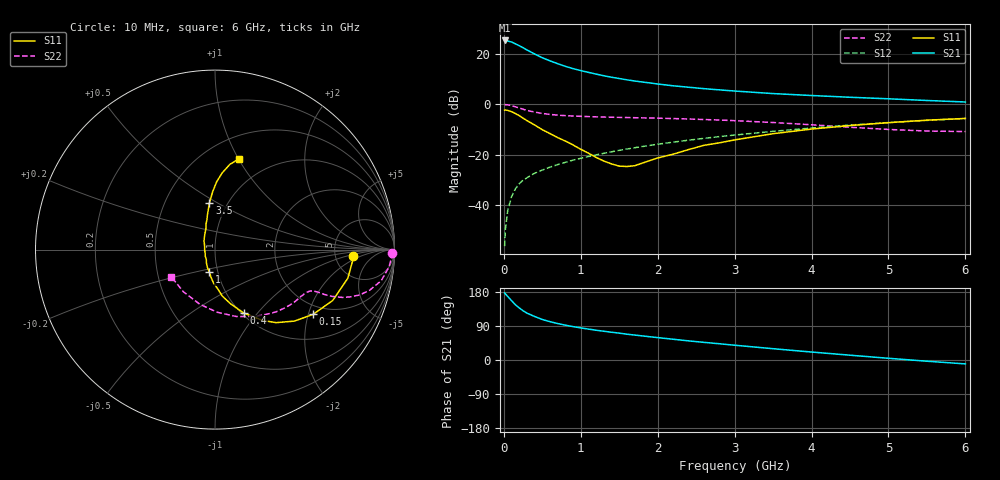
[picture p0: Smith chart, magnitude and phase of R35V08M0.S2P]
! SIEMENS Small Signal Semiconductors
! BFR181
! Si NPN RF Bipolar Junction Transistor in SOT23
! VCE = 5 V  IC = 8 mA
! Common Emitter S-Parameters:  May  1996
# GHz  S  MA  R  50
!  f  S11  S21  S12  S22
! GHz  MAG  ANG  MAG  ANG  MAG  ANG  MAG  ANG
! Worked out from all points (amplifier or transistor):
!   36 points, 10 MHz to 6 GHz, reference 50 ohm
!   highest |S21| = 25.4 dB at 10 MHz (marker M1)
!   |S21| within 3 dB of that: start of sweep to 256 MHz
!   unconditionally stable (mu >= 1): 925.5 MHz to 2.78 GHz
!   at 250 MHz: K = 0.54, MSG = 26.4 dB, |S12| = -30.2 dB
!   at 1.4 GHz: K = 1.05, MAG = 13.4 dB, |S12| = -18.9 dB
!   at 6 GHz: K = 0.86, MSG = 3.3 dB, |S12| = -5.7 dB
!   S11 on the Smith chart (normalised r, x): 10 MHz: 7.45, -1.22; 150 MHz: 1.70, -2.15; 400 MHz: 1.02, -0.85; 1 GHz: 0.91, -0.23; 3.5 GHz: 0.82, +0.46; 6 GHz: 0.72, +1.01
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0.01  0.769 -2.5  18.68 177.0  0.0015 92.8  0.9884 -1.0
0.02  0.7693 -4.7  18.54 174.5  0.0032 85.1  0.9853 -2.3
0.05  0.7569 -12.2  18.2 167.8  0.0076 84.9  0.9749 -5.6
0.1  0.7144 -23.4  17.39 156.6  0.0145 79.6  0.9423 -10.6
0.15  0.6551 -33.4  16.02 145.8  0.0208 74.3  0.891 -14.7
0.2  0.5953 -42.0  14.69 137.5  0.0263 71.7  0.845 -17.4
0.25  0.5306 -50.1  13.38 129.9  0.0309 68.9  0.7977 -19.3
0.3  0.4745 -56.2  12.09 123.7  0.0345 68.8  0.7572 -20.6
0.4  0.3881 -65.6  10.05 114.9  0.0424 67.1  0.7011 -21.8
0.5  0.3124 -74.2  8.446 106.9  0.0491 66.9  0.6584 -22.3
0.6  0.2616 -81.1  7.334 101.1  0.0562 67.5  0.6287 -22.4
0.7  0.2175 -86.3  6.441 96.2  0.063 68.0  0.6093 -22.6
0.8  0.1854 -92.8  5.703 91.9  0.0701 67.8  0.5947 -22.8
1  0.1273 -104.6  4.691 84.7  0.0841 68.3  0.5758 -23.7
1.1  0.1064 -113.8  4.323 81.6  0.0913 68.4  0.5692 -24.4
1.3  0.0742 -130.5  3.702 75.9  0.1061 68.0  0.5574 -25.8
1.6  0.0578 -179.6  3.071 68.1  0.1289 67.5  0.545 -28.6
2.2  0.1015 124.3  2.338 54.8  0.1765 64.4  0.5205 -36.1
3.5  0.2603 97.0  1.636 29.8  0.2898 54.4  0.4344 -59.1
4.5  0.378 88.6  1.382 12.7  0.3858 43.8  0.3495 -87.9
5.5  0.4832 80.0  1.192 -3.2  0.479 31.1  0.2937 -126.6
6  0.5237 75.1  1.112 -10.3  0.5215 24.3  0.2871 -148.4
